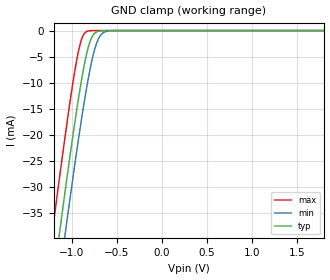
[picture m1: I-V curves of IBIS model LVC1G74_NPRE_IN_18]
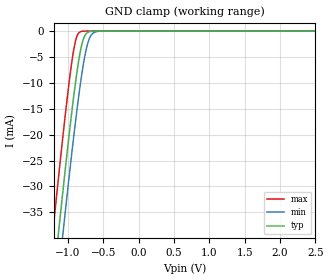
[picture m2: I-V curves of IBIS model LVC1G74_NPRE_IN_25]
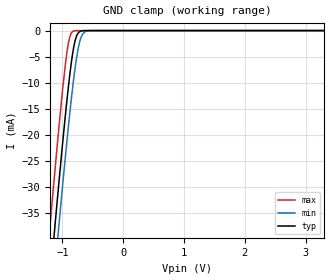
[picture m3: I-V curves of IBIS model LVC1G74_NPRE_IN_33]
| TEXAS INSTRUMENTS INCORPORATED
| Standard Linear and Logic Group
| IBIS Model of SN74LVC1G74
| SINGLE POSITIVE-EDGE-TRIGGERED D-TYPE FLIP FLOP WITH CLEAR AND PRESET
| This file contains package information for the following:
|  SSOP 8-pin (DCT) package as [Component] LVC1G74_DCT
|  VSSOP 8-pin (DCU) package as [Component] LVC1G74_DCU
|  8-pin RES package as [Component] LVC1G74_RSE
|  8-pin (DQE) package as [Component] LVC1G74_DQE
| This device can be powered at the following Vccs:
|  1.8 volt Vcc
|  2.5 volt Vcc
|  3.3 volt Vcc
|  5 volt Vcc
| This file provides unique models under the [Model Selector] for each Vcc.
| For operation at a specific Vcc, select the appropriate model after each
| [Model Selector] keyword.
[IBIS Ver]   3.2
[Comment char]  |_char
[File Name]   sn74lvc1g74.ibs
[File Rev]   1.1 | d_die
[Date]   July 25, 2019
[Source]   Data created from TI-SPICE simulations at TI-SLL.
[Notes]   The following is an IBIS list for the LVC1G74.
   Please contact sllibis@ti.com with questions and
   comments concerning SLL IBIS models.
   - Power-clamp data has been deleted since there is no
   power-clamp diode in the device. s
   - Due to the fact that the device is 5-V input/output
   tolerant, the pullup data has some non-monotonic warnings.
   - Due to the fact that the Device is 5.5-V Input tolarent,
   the pulldown model has some Non-Monotonic Warnings.
[Disclaimer] Property of Texas Instruments Incorporated.  Unauthorized
   reproduction and/or distribution is strictly prohibited.
   This product is protected under copyright law.
   Created  2019, (C) Copyright  2019, Texas Instruments
   Incorporated, All Rights Reserved
   UNLESS THERE IS A SIGNED, WRITTEN AGREEMENT TO THE
   CONTRARY, TEXAS INSTRUMENTS (TI) IS PROVIDING THE IBIS
   MODELS  AND WITHOUT ANY WARRANTY, EXPRESSED OR
   IMPLIED.  TI assumes no liability for:
   1) the accuracy of the IBIS models provided to your
   company;
   2) the proper functioning of these IBIS Models in your
   design or for any resulting applications; or
   3) infringement of patents, copyrights or intellectual
   property rights resulting from your use of these IBIS
   models.
   TI provides IBIS Models as a service to our customers.
   You and your company shall not distribute, sell or give
   these models to anyone else without prior written
   permission from TI.
   TI reserves the right to make changes to our products or
   to discontinue any semiconductor product or service
   without notice, and advises our customers to obtain the
   latest version of relevant information to verify, before
   placing orders, that the information being relied on is
   current.
   Please be aware that your receipt and use of the IBIS
   information provided shall serve as acceptance of these
   terms and conditions.  If you do not accept these terms,
   you should return or destroy the IBIS models and any
   other accompanying information immediately.
| Component LVC1G74_DCT 8-pin SOT
[Component]   LVC1G74_DCT
[Manufacturer]   Texas Instruments, Inc.
[Package]
|   typ   min   max
R_pkg   2.900e-02   2.800e-02   3.100e-02
L_pkg   1.796e-09   1.666e-09   1.924e-09
C_pkg   2.310e-13   2.210e-13   2.420e-13
[Pin]   signal_name   model_name   R_pin   L_pin   C_pin
1   CLK   LVC1G74_IN   3.100e-02   1.894e-09   2.230e-13
2   D   LVC1G74_IN   2.800e-02   1.697e-09   2.370e-13
3   NQ   LVC1G74_OUT   3.000e-02   1.722e-09   2.390e-13
4   GND   GND   3.000e-02   1.861e-09   2.210e-13
5   Q   LVC1G74_OUT   2.800e-02   1.924e-09   2.280e-13
6   NCLR   LVC1G74_NCLR_IN   2.900e-02   1.736e-09   2.420e-13
7   NPRE   LVC1G74_NPRE_IN   2.800e-02   1.666e-09   2.360e-13
8   VCC   POWER   3.000e-02   1.871e-09   2.220e-13
| Component LVC1G74_DCU 8-pin SOT
[Component]   LVC1G74_DCU
[Manufacturer]   Texas Instruments, Inc.
[Package]
|   typ   min   max
R_pkg   2.600e-02   2.300e-02   3.800e-02
L_pkg   1.394e-09   1.066e-09   2.046e-09
C_pkg   2.590e-13   2.150e-13   3.720e-13
[Pin]   signal_name   model_name   R_pin   L_pin   C_pin
1   CLK   LVC1G74_IN   2.400e-02   1.520e-09   2.710e-13
2   D   LVC1G74_IN   2.300e-02   1.112e-09   2.180e-13
3   NQ   LVC1G74_OUT   2.300e-02   1.070e-09   2.170e-13
4   GND   GND   2.700e-02   2.046e-09   3.720e-13
5   Q   LVC1G74_OUT   2.700e-02   1.542e-09   2.730e-13
6   NCLR   LVC1G74_IN   2.300e-02   1.100e-09   2.240e-13
7   NPRE   LVC1G74_IN   2.300e-02   1.066e-09   2.150e-13
8   VCC   POWER   3.800e-02   1.696e-09   2.800e-13
| Component LVC1G74_PW 8-PIN DQE
[Component]   LVC1G74_DQE
[Manufacturer]   Texas Instruments, Inc.
[Package]
|   typ   min   max
R_pkg   4.041e-02   2.609e-02   5.397e-02
L_pkg   3.575e-10   2.969e-10   4.398e-10
C_pkg   5.781e-14   5.009e-14   6.768e-14
[Pin]   signal_name   model_name   R_pin   L_pin   C_pin
1   CLK   LVC1G74_IN   NA   NA   NA
2   D   LVC1G74_IN   NA   NA   NA
3   NQ   LVC1G74_OUT   NA   NA   NA
4   GND   GND   NA   NA   NA
5   Q   LVC1G74_OUT   NA   NA   NA
6   NCLR   LVC1G74_IN   NA   NA   NA
7   NPRE   LVC1G74_IN   NA   NA   NA
8   VCC   POWER   NA   NA   NA
| Component LVC1G74_RSE
[Component]   LVC1G74_RSE
[Manufacturer]   Texas Instruments, Inc.
[Package]
|   typ   min   max
R_pkg   0.07384   0.06172   0.08697
L_pkg   0.51021nH   0.40726nH   0.62174nH
C_pkg   0.18219pF   0.17417pF   0.19566pF
[Pin]   signal_name   model_name   R_pin   L_pin   C_pin
1   CLK   LVC1G74_IN   NA   NA   NA
2   D   LVC1G74_IN   NA   NA   NA
3   NQ   LVC1G74_OUT   NA   NA   NA
4   GND   GND   NA   NA   NA
5   Q   LVC1G74_OUT   NA   NA   NA
6   NCLR   LVC1G74_IN   NA   NA   NA
7   NPRE   LVC1G74_IN   NA   NA   NA
8   VCC   POWER   NA   NA   NA
| Model LVC1G74_NPRE_IN
[Model Selector]   LVC1G74_NPRE_IN
LVC1G74_NPRE_IN_18   1.8 volt Vcc
LVC1G74_NPRE_IN_25   2.5 volt Vcc
LVC1G74_NPRE_IN_33   3.3 volt Vcc
LVC1G74_NPRE_IN_50   5 volt Vcc
| Model LVC1G74_NCLR_IN
[Model Selector]   LVC1G74_NCLR_IN
LVC1G74_NCLR_IN_18   1.8 volt Vcc
LVC1G74_NCLR_IN_25   2.5 volt Vcc
LVC1G74_NCLR_IN_33   3.3 volt Vcc
LVC1G74_NCLR_IN_50   5 volt Vcc
| Model LVC1G74_IN
[Model Selector]   LVC1G74_IN
LVC1G74_IN_18   1.8 volt Vcc
LVC1G74_IN_25   2.5 volt Vcc
LVC1G74_IN_33   3.3 volt Vcc
LVC1G74_IN_50   5 volt Vcc
| Model LVC1G74_OUT
[Model Selector]   LVC1G74_OUT
LVC1G74_OUT_18   1.8 volt Vcc
LVC1G74_OUT_25   2.5 volt Vcc
LVC1G74_OUT_33   3.3 volt Vcc
LVC1G74_OUT_50   5 volt Vcc
| Models and submodels in the file (16): LVC1G74_NPRE_IN_18 (Input), LVC1G74_NPRE_IN_25 (Input), LVC1G74_NPRE_IN_33 (Input), LVC1G74_NPRE_IN_50 (Input), LVC1G74_NCLR_IN_18 (Input), LVC1G74_NCLR_IN_25 (Input), LVC1G74_NCLR_IN_33 (Input), LVC1G74_NCLR_IN_50 (Input), LVC1G74_IN_18 (Input), LVC1G74_IN_25 (Input), LVC1G74_IN_33 (Input), LVC1G74_IN_50 (Input), LVC1G74_OUT_18 (Output), LVC1G74_OUT_25 (Output), LVC1G74_OUT_33 (Output), LVC1G74_OUT_50 (Output)
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[Model]   LVC1G74_NPRE_IN_18
Model_type  Input
Vinl=0.5775
Vinh=1.2675
| variable   typ   min   max
C_comp   3.50pF   2.98pF   4.30pF
[Temperature Range]   40   100   -40
| Ambient temperature   25   85   -40
[Voltage range]   1.8   1.65   1.95
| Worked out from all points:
|   GND clamp passes 1 mA (typ) near -0.77 V on its own axis
[GND Clamp]
| LVC1G74_NPRE_IN_18
|   Voltage   I(typ)   I(min)   I(max)
-5.5V     -655.2mA   -662.2mA   -646.6mA
-1.215V   -49.6mA    -57.88mA   -38.96mA
-1.135V   -39.07mA   -47.36mA   -28.42mA
-1.075V   -31.35mA   -39.6mA    -20.75mA
-1.055V   -28.82mA   -37.05mA   -18.27mA
-955mV    -16.68mA   -24.66mA   -6.874mA
-885mV    -9.098mA   -16.55mA   -1.486mA
-825mV    -3.922mA   -10.26mA   -137.1uA
-780mV    -1.472mA   -6.227mA   -17.15uA
-715mV    -205.4uA   -2.128mA   -808.5nA
-650mV    -22.01uA   -443.9uA   -37.93nA
1.8V      3.326pA    6.142pA    3.026pA
[Model]   LVC1G74_NPRE_IN_25
Model_type  Input
Vinl=0.7
Vinh=1.7
| variable   typ   min   max
C_comp   3.43pF   2.80pF   4.40pF
[Temperature Range]   40   100   -40
| Ambient temperature   25   85   -40
[Voltage range]   2.5   2.3   2.7
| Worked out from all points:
|   GND clamp passes 1 mA (typ) near -0.77 V on its own axis
[GND Clamp]
| LVC1G74_NPRE_IN_25
|   Voltage   I(typ)   I(min)   I(max)
-5.5V     -655.2mA   -662.2mA   -646.6mA
-1.215V   -49.6mA    -57.88mA   -38.96mA
-1.14V    -39.72mA   -48.01mA   -29.07mA
-1.12V    -37.12mA   -45.41mA   -26.48mA
-1.08V    -31.98mA   -40.25mA   -21.38mA
-1.06V    -29.44mA   -37.69mA   -18.89mA
-960mV    -17.26mA   -25.26mA   -7.377mA
-890mV    -9.597mA   -17.1mA    -1.734mA
-785mV    -1.671mA   -6.635mA   -21.67uA
-720mV    -242.5uA   -2.354mA   -1.023uA
-650mV    -22.01uA   -443.9uA   -37.93nA
2.5V      4.713pA    7.577pA    4.389pA
[Model]   LVC1G74_NPRE_IN_33
Model_type  Input
Vinl=0.8
Vinh=2.0
| variable   typ   min   max
C_comp   3.34pF   2.69pF   4.33pF
[Temperature Range]   40   100   -40
| Ambient temperature   25   85   -40
[Voltage range]   3.3   3   3.6
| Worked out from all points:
|   GND clamp passes 1 mA (typ) near -0.77 V on its own axis
[GND Clamp]
| LVC1G74_NPRE_IN_33
|   Voltage   I(typ)   I(min)   I(max)
-5.5V     -655.2mA   -662.2mA   -646.6mA
-1.225V   -50.93mA   -59.21mA   -40.3mA
-1.145V   -40.37mA   -48.66mA   -29.72mA
-1.12V    -37.12mA   -45.41mA   -26.48mA
-1.08V    -31.98mA   -40.25mA   -21.38mA
-1.06V    -29.44mA   -37.69mA   -18.89mA
-965mV    -17.84mA   -25.87mA   -7.89mA
-885mV    -9.098mA   -16.55mA   -1.486mA
-780mV    -1.472mA   -6.227mA   -17.15uA
-715mV    -205.4uA   -2.128mA   -808.5nA
-640mV    -15.53uA   -338.1uA   -23.69nA
3.3V      6.304pA    9.258pA    5.93pA
